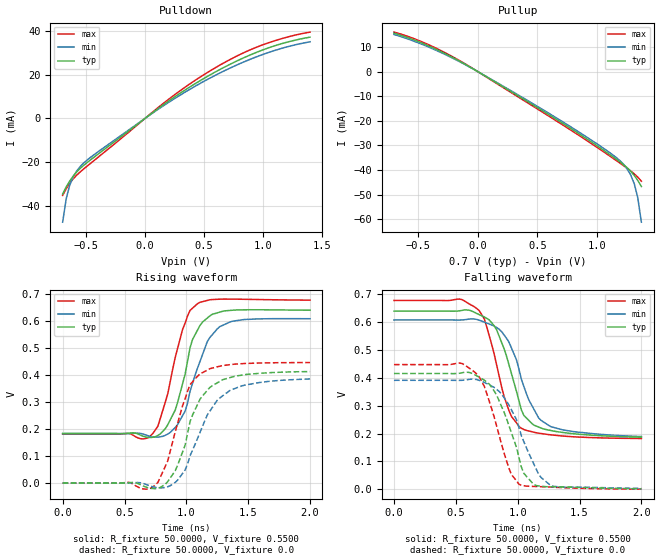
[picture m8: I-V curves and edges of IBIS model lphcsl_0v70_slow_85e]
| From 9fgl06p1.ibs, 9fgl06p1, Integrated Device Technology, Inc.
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[Model]   lphcsl_0v70_slow_85e
Model_type Output
Polarity   Inverting
Enable   Active-High
Vmeas =  0.4000V
Cref =   2.0000pF
Rref =   0.0
Vref =   0.4000V
C_comp   1.1000pF   1.0000pF   1.2000pF
[Temperature Range]   25.0000   85.0000   -40.0000
[Voltage Range]   0.7000V   0.6700V   0.7400V
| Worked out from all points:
|   slope of the pulldown table from 0 to 0.105 V, typ, clamps not added: 24.6 ohm
|   slope of the pullup table from 0 to 0.105 V, typ, clamps not added: 34.4 ohm
|   rising waveform, R_fixture 50.0000, V_fixture 0.5500: 20-80 % time 157ps typ, 178ps min, 161ps max; typ from 0.184 V to 0.641 V
|   rising waveform, R_fixture 50.0000, V_fixture 0.0: 20-80 % time 202ps typ, 240ps min, 170ps max; typ from 0 V to 0.413 V
|   falling waveform, R_fixture 50.0000, V_fixture 0.5500: 20-80 % time 187ps typ, 215ps min, 178ps max; typ from 0.639 V to 0.187 V
|   falling waveform, R_fixture 50.0000, V_fixture 0.0: 20-80 % time 192ps typ, 228ps min, 180ps max; typ from 0.415 V to 0.002 V
[Pulldown]
|Voltage   I(typ)   I(min)   I(max)
-700mV    -34.6mA    -47.52mA   -35.24mA
-670mV    -31.39mA   -36.87mA   -32.23mA
-640mV    -28.69mA   -30.58mA   -29.71mA
-610mV    -26.4mA    -26.67mA   -27.65mA
-550mV    -22.86mA   -21.99mA   -24.47mA
-430mV    -17.63mA   -16.5mA    -19.15mA
200mV     7.926mA    7.321mA    8.744mA
560mV     20.14mA    18.69mA    22.01mA
770mV     26.03mA    24.22mA    28.28mA
980mV     30.93mA    28.85mA    33.27mA
1.19V     34.64mA    32.5mA     36.93mA
1.4V      37.16mA    35.04mA    39.47mA
[Pullup]
|Voltage   I(typ)   I(min)   I(max)
-700mV    15.57mA    15.04mA    16.02mA
-430mV    10.81mA    10.36mA    11.32mA
-130mV    3.627mA    3.457mA    3.841mA
590mV     -17.35mA   -16.8mA    -17.95mA
890mV     -26.63mA   -25.92mA   -27.3mA
1.13V     -34.56mA   -33.83mA   -35.16mA
1.22V     -37.82mA   -37.66mA   -38.23mA
1.25V     -39.06mA   -39.49mA   -39.29mA
1.28V     -40.5mA    -41.94mA   -40.38mA
1.31V     -42.21mA   -45.54mA   -41.56mA
1.34V     -44.27mA   -51.36mA   -42.91mA
1.37V     -46.73mA   -61.22mA   -44.56mA
[Ramp]
| variable   typ   min   max
dV/dt_r  0.2480/0.2224n   0.2316/0.2472n   0.2681/0.1864n
dV/dt_f  0.2762/0.2214n   0.2549/0.2470n   0.3031/0.1879n
R_load = 50.0000
[Rising Waveform]
R_fixture= 50.0000
V_fixture= 0.5500
V_fixture_min= 0.5200
V_fixture_max= 0.5800
|time   V(typ)   V(min)   V(max)
0s        184mV      183.2mV    181.4mV
710ps     168.8mV    173mV      175.2mV
770ps     176.8mV    170.4mV    211mV
930ps     300.1mV    217.7mV    500.8mV
990ps     403.8mV    267mV      592.6mV
1.03ns    502mV      340.4mV    640.2mV
1.11ns    584.1mV    450.6mV    670.1mV
1.19ns    619.7mV    539.6mV    679.4mV
1.35ns    639.8mV    596.6mV    681.9mV
2ns       640.8mV    609.2mV    678.1mV
[Rising Waveform]
R_fixture= 50.0000
V_fixture= 0.0
V_fixture_min= 0.0
V_fixture_max= 0.0
|time   V(typ)   V(min)   V(max)
0s        0V         0V         0V
690ps     -17.28mV   -7.689mV   -22.36mV
790ps     -15.93mV   -17.58mV   22.34mV
910ps     45.82mV    2.628mV    190.4mV
990ps     141mV      48.89mV    312.7mV
1.03ns    228.1mV    101.4mV    364.9mV
1.11ns    310.6mV    187.5mV    404.4mV
1.25ns    371.6mV    307.3mV    431mV
1.35ns    390.6mV    342.7mV    438.8mV
2ns       413.3mV    386mV      446.8mV
[Falling Waveform]
R_fixture= 50.0000
V_fixture= 0.5500
V_fixture_min= 0.5200
V_fixture_max= 0.5800
|time   V(typ)   V(min)   V(max)
0s        638.8mV    607.1mV    677mV
530ps     639.8mV    606.8mV    682mV
690ps     626mV      606.1mV    640.1mV
730ps     617.9mV    599.4mV    611mV
830ps     571.9mV    579.8mV    445.9mV
930ps     445.9mV    527.2mV    282mV
1.03ns    284.8mV    394.3mV    218.9mV
1.17ns    223.2mV    255.7mV    201.3mV
1.27ns    210.8mV    224.4mV    195.2mV
2ns       186.9mV    189.2mV    182.3mV
[Falling Waveform]
R_fixture= 50.0000
V_fixture= 0.0
V_fixture_min= 0.0
V_fixture_max= 0.0
|time   V(typ)   V(min)   V(max)
0s        415.1mV    390.8mV    447.1mV
530ps     416.1mV    390.5mV    452.7mV
650ps     411.6mV    394.8mV    421.3mV
730ps     391.3mV    383.2mV    369.4mV
830ps     337.9mV    358.5mV    226.7mV
930ps     227.7mV    301.8mV    75.09mV
1.01ns    115.3mV    222.7mV    18.35mV
1.13ns    17.33mV    91.39mV    10.45mV
1.27ns    9.268mV    12.74mV    8.046mV
2ns       1.891mV    3.2mV      630.1uV
